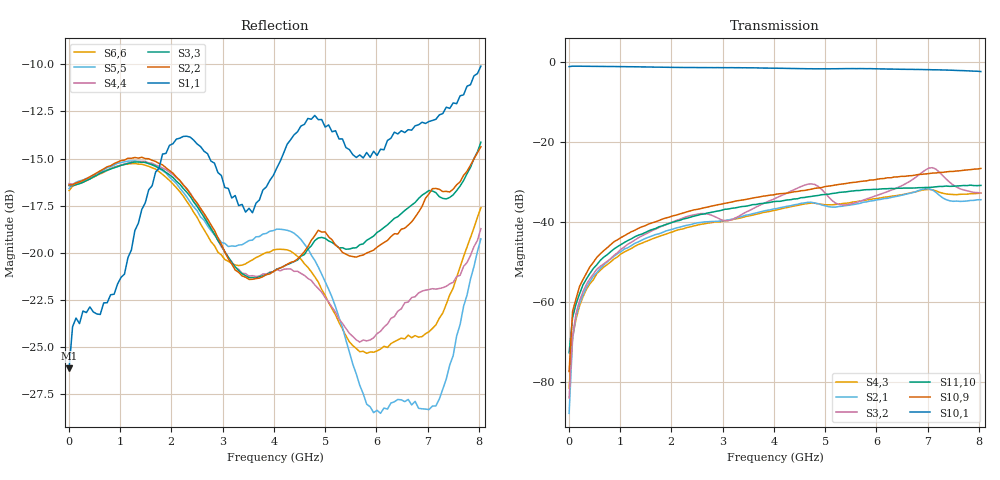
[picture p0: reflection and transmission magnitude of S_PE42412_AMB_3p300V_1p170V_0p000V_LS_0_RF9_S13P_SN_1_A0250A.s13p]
! Device ID: PE42412
! File Path: z:\PE42412\TE_GND_Post_Char_S-Param\All Parts\AMB\3p300\LS_0_RF9\PE42412_AMB_3p300V_1p170V_0p000V_LS_0_RF9_S13P_SN_1_A0250A.s13p
! Serial: 1
! Lot: A0250A
! Temp: AMB
! VDD: 3.300
! VSS: 0.000
! Control_Hi: 1.170
! Control_Lo: 0.000
! Logic State: LS_0_RF9
! Port 1:
! Port 2:
! Port 3:
! Port 4:
! Port 5:
! Port 6:
! Port 7:
! Port 8:
! Port 9:
! Port 10:
! Port 11:
! Port 12:
! Port 13:
! ThroughPath:1-10
! IDD: 0.0001063701
! ISS/IDD2: 1.67e-008
! IDMM3/IDD3: -1.572e-007
! Comment:
#  Hz  S  RI  R  50
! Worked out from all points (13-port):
!   120 points, 10 MHz to 8.037 GHz, reference 50 ohm
!   strongest paths, dB at 10 MHz, 2.034 GHz, 4.057 GHz, 6.08 GHz, 8.037 GHz:
!     S10,1: -1.0, -1.2, -1.4, -1.6, -2.3
!     S10,9: -77.5, -38.4, -33.0, -29.1, -26.6
!     S11,10: -72.7, -40.0, -34.8, -31.7, -30.8
!     S3,2: -84.1, -40.0, -33.9, -33.0, -32.7
!     S2,1: -87.9, -41.8, -36.6, -34.3, -34.4
!     S4,3: -81.6, -42.4, -37.0, -34.0, -32.8
!   lowest |S11| = -26.1 dB at 10 MHz (marker M1), VSWR 1.10, Z = 54.3 - j2.93 ohm
!   |S11| at or under -10 dB: start of sweep to end of sweep
